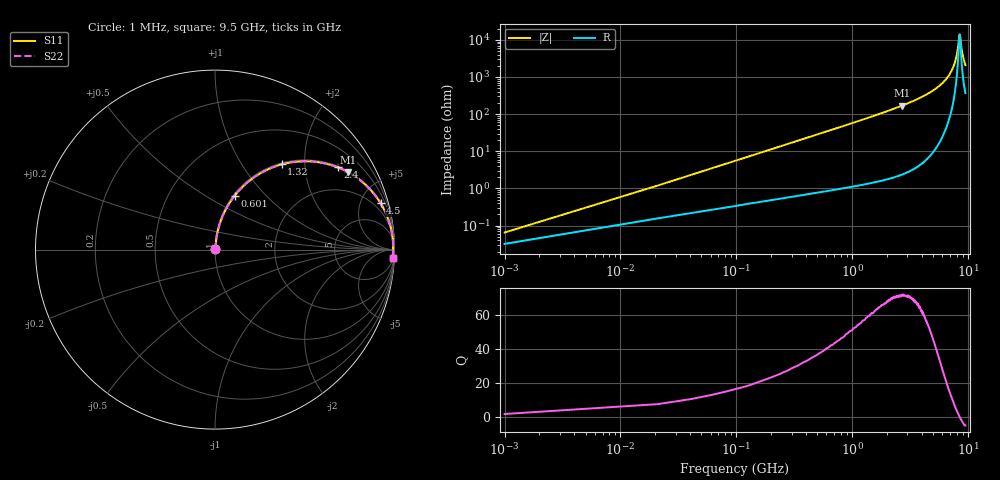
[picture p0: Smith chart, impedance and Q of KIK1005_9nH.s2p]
!version-3
!date-01.2023
!Series
# MHz S RI R 50
!Freq ReS11 ImS11 ReS21 ImS21 ReS12 ImS12 ReS22 ImS22
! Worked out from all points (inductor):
!   476 points, 1 MHz to 9.5 GHz, reference 50 ohm
!   read as one part in series: L = 9 nH near 41 MHz
!   highest Q = 72 at 2.7 GHz (marker M1), where L = 10 nH
!   self-resonance near 8.48 GHz
!   S11 on the Smith chart (normalised r, x): 1 MHz: 1.00, +0.00; 601 MHz: 1.02, +0.68; 1.32 GHz: 1.03, +1.53; 2.4 GHz: 1.04, +2.95; 4.5 GHz: 1.13, +7.08; 9.5 GHz: 8, -41
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1  0.000342 0.000565  0.9997 -0.000565  0.9997 -0.000565  0.000342 0.000565
61  0.00384 0.0343  0.9962 -0.0343  0.9962 -0.0343  0.00384 0.0343
81  0.00514 0.0454  0.9949 -0.0454  0.9949 -0.0454  0.00514 0.0454
121  0.00835 0.0676  0.9916 -0.0676  0.9916 -0.0676  0.00835 0.0676
201  0.0174 0.1112  0.9826 -0.1112  0.9826 -0.1112  0.0174 0.1112
301  0.0336 0.1637  0.9664 -0.1637  0.9664 -0.1637  0.0336 0.1637
601  0.1104 0.3013  0.8896 -0.3013  0.8896 -0.3013  0.1104 0.3013
1320  0.3717 0.4748  0.6283 -0.4748  0.6283 -0.4748  0.3717 0.4748
1600  0.469 0.4912  0.531 -0.4912  0.531 -0.4912  0.469 0.4912
2400  0.683 0.4583  0.317 -0.4583  0.317 -0.4583  0.683 0.4583
2700  0.7399 0.4318  0.2601 -0.4318  0.2601 -0.4318  0.7399 0.4318
3180  0.8107 0.3847  0.1893 -0.3847  0.1893 -0.3847  0.8107 0.3847
4500  0.9221 0.259  0.0779 -0.259  0.0779 -0.259  0.9221 0.259
4760  0.935 0.2367  0.065 -0.2367  0.065 -0.2367  0.935 0.2367
6340  0.98 0.12  0.02 -0.12  0.02 -0.12  0.98 0.12
7300  0.9902 0.0619  0.00983 -0.0619  0.00983 -0.0619  0.9902 0.0619
7920  0.9927 0.0284  0.00732 -0.0284  0.00732 -0.0284  0.9927 0.0284
8160  0.993 0.0161  0.00701 -0.0161  0.00701 -0.0161  0.993 0.0161
8420  0.993 0.00321  0.00704 -0.00321  0.00704 -0.00321  0.993 0.00321
8500  0.9929 -0.000671  0.00712 0.000671  0.00712 0.000671  0.9929 -0.000671
8960  0.9919 -0.0223  0.00815 0.0223  0.00815 0.0223  0.9919 -0.0223
9500  0.9895 -0.0461  0.0105 0.0461  0.0105 0.0461  0.9895 -0.0461
